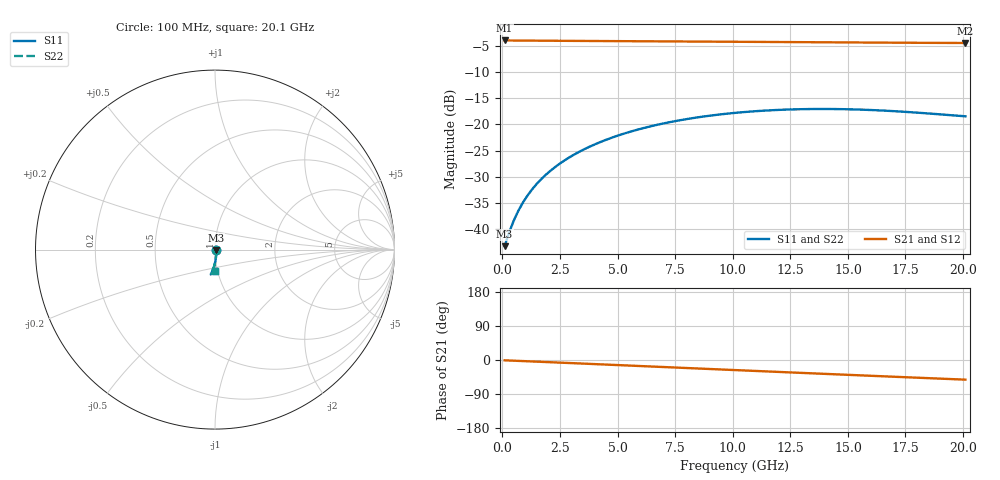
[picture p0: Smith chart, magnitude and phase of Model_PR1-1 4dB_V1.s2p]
!version-1
!date-07.2020
!Series
#	GHZ S RI R 50.0
!	FREQ.GHZ	S11RE	S11IM	S21RE	S21IM	S12RE	S12IM	S22RE	S22IM
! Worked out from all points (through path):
!   101 points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, 100 MHz to 20.1 GHz, reference 50 ohm
!   highest |S21| = -3.94 dB at 100 MHz (marker M1); lowest = -4.4 dB at 20.1 GHz (marker M2)
!   group delay of S21, straight-line fit = 7.12 ps
!   lowest |S11| = -43.3 dB at 100 MHz (marker M3), VSWR 1.01, Z = 50.5 - j0.424 ohm
!   |S11| at or under -10 dB: start of sweep to end of sweep
!   |S22| runs from -43.3 to -17.0 dB; largest |S21 - S12| = 0
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0.1  0.00542 -0.0042  0.6351 -0.00928  0.6351 -0.00928  0.00542 -0.0042
0.3  0.00571 -0.00736  0.6346 -0.0148  0.6346 -0.0148  0.00571 -0.00736
0.5  0.00594 -0.0105  0.634 -0.0203  0.634 -0.0203  0.00594 -0.0105
0.7  0.00611 -0.0137  0.6334 -0.0259  0.6334 -0.0259  0.00611 -0.0137
0.9  0.00622 -0.0169  0.6328 -0.0314  0.6328 -0.0314  0.00622 -0.0169
1.1  0.00628 -0.02  0.632 -0.037  0.632 -0.037  0.00628 -0.02
1.3  0.00628 -0.0232  0.6313 -0.0425  0.6313 -0.0425  0.00628 -0.0232
1.7  0.00613 -0.0295  0.6296 -0.0536  0.6296 -0.0536  0.00613 -0.0295
2.3  0.00556 -0.0389  0.6268 -0.0703  0.6268 -0.0703  0.00556 -0.0389
2.9  0.00461 -0.048  0.6236 -0.087  0.6236 -0.087  0.00461 -0.048
3.5  0.00334 -0.057  0.6199 -0.1036  0.6199 -0.1036  0.00334 -0.057
4.3  0.00123 -0.0684  0.6143 -0.1256  0.6143 -0.1256  0.00123 -0.0684
5.1  -0.00123 -0.0793  0.608 -0.1474  0.608 -0.1474  -0.00123 -0.0793
5.9  -0.00395 -0.0894  0.6009 -0.1689  0.6009 -0.1689  -0.00395 -0.0894
6.9  -0.00753 -0.1009  0.591 -0.1954  0.591 -0.1954  -0.00753 -0.1009
8.5  -0.0132 -0.1162  0.5728 -0.2367  0.5728 -0.2367  -0.0132 -0.1162
10.1  -0.0183 -0.1276  0.5518 -0.2761  0.5518 -0.2761  -0.0183 -0.1276
11.7  -0.022 -0.1349  0.5281 -0.3136  0.5281 -0.3136  -0.022 -0.1349
13.5  -0.0238 -0.1383  0.4985 -0.3531  0.4985 -0.3531  -0.0238 -0.1383
15.1  -0.0229 -0.1375  0.47 -0.3858  0.47 -0.3858  -0.0229 -0.1375
16.9  -0.0184 -0.133  0.4358 -0.4197  0.4358 -0.4197  -0.0184 -0.133
20.1  -0.000152 -0.1196  0.3711 -0.4726  0.3711 -0.4726  -0.000152 -0.1196
